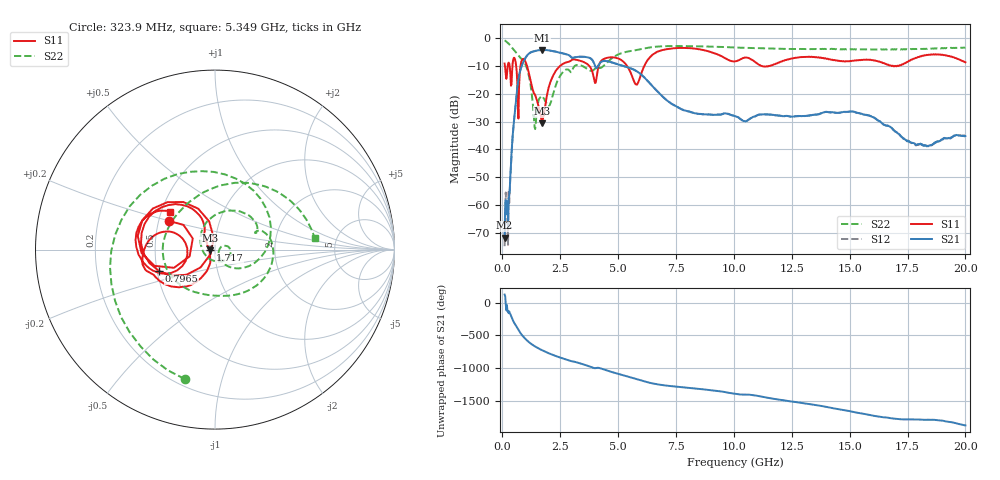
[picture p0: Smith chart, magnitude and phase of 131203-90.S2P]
!  2-Port S-parameters saved by WinCal
! VAR MeasName=S-Parameters (CALIBRATED_DATA) read from VNA (N5244A)
! VAR MeasDate=4/4/2013 3:59:26 PM
! VAR NAME=131203-90
! VAR FILENAME=131203-90.S2P
! VAR DATE=4/4/2013 3:59:26 PM
! VAR PHYS_PORTS=1,2
# Hz S MA R 50
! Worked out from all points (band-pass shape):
!   801 points, 100 MHz to 20 GHz, reference 50 ohm
!   highest |S21| = -4.36 dB at 1.717 GHz (marker M1); lowest = -71.6 dB at 100 MHz (marker M2)
!   |S21| within 3 dB of the highest: 988 MHz to 3.806 GHz (2.818 GHz wide, 118 % of centre)
!   lowest |S11| = -30.6 dB at 1.717 GHz (marker M3), VSWR 1.06, Z = 47.2 - j0.399 ohm
!   |S11| at or under -10 dB: 1.064 GHz to 2.505 GHz (1.441 GHz wide, 80.7 % of centre); 3.749 GHz to 4.166 GHz (417.3 MHz wide, 10.5 % of centre); 5.379 GHz to 6.139 GHz (759.4 MHz wide, 13.2 % of centre)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
!   |S22| runs from -32.7 to -1.0 dB; largest |S21 - S12| = 0.0032
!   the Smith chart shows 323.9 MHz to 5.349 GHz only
!   S11 on the Smith chart (normalised r, x): 323.9 MHz: 0.57, +0.20; 796.5 MHz: 0.51, -0.14; 1.717 GHz: 0.94, -0.01; 5.349 GHz: 0.55, +0.26
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1e8  0.3459 153.0  0.0002637 120.9  0.0001853 145.4  0.8957 -32.7
3.23875e8  0.2993 147.9  0.00199 -165.4  0.001939 -160.6  0.74 -103.3
5.4775e8  0.4148 146.4  0.05007 32.6  0.05004 32.8  0.5783 -179.1
7.965e8  0.3335 -158.9  0.2789 -109.5  0.2796 -109.4  0.4329 90.9
1.020375e9  0.3581 136.1  0.4501 160.7  0.4511 160.7  0.3178 13.7
1.269125e9  0.137 114.8  0.5568 87.1  0.559 87.2  0.1024 -55.7
1.418375e9  0.094 129.7  0.5796 53.1  0.581 53.1  0.02313 -8.6
1.716875e9  0.02953 -171.8  0.6052 -3.7  0.6067 -3.7  0.09047 -21.4
2.313875e9  0.2572 -127.2  0.5638 -92.0  0.5656 -92.0  0.1415 116.5
2.811375e9  0.3661 -156.0  0.4996 -151.1  0.5012 -151.2  0.2715 34.7
3.43325e9  0.3787 174.4  0.4575 149.3  0.4583 149.1  0.3156 -31.1
4.12975e9  0.2759 -152.0  0.3072 90.5  0.3086 90.3  0.2912 172.3
4.62725e9  0.4459 173.3  0.3724 36.6  0.3741 36.2  0.3952 70.5
5.348625e9  0.3298 140.0  0.3023 -35.3  0.303 -35.6  0.5591 6.6
5.796375e9  0.1444 170.0  0.2532 -82.3  0.2536 -82.6  0.6039 -17.2
6.741625e9  0.5727 176.2  0.1053 -163.2  0.106 -163.6  0.6961 -57.1
8.383375e9  0.6339 124.1  0.04405 133.6  0.04392 133.0  0.7029 -109.7
1.005e10  0.3789 106.6  0.03959 55.9  0.03941 55.7  0.6714 -147.8
1.338325e10  0.4545 92.3  0.04135 -107.5  0.04116 -107.0  0.6267 162.0
1.669162e10  0.324 70.7  0.02628 50.2  0.02639 50.4  0.6161 127.5
1.788562e10  0.4376 81.7  0.01217 25.8  0.01184 26.1  0.6284 118.2
2e10  0.3643 35.7  0.01745 -64.7  0.01724 -66.0  0.667 102.1
